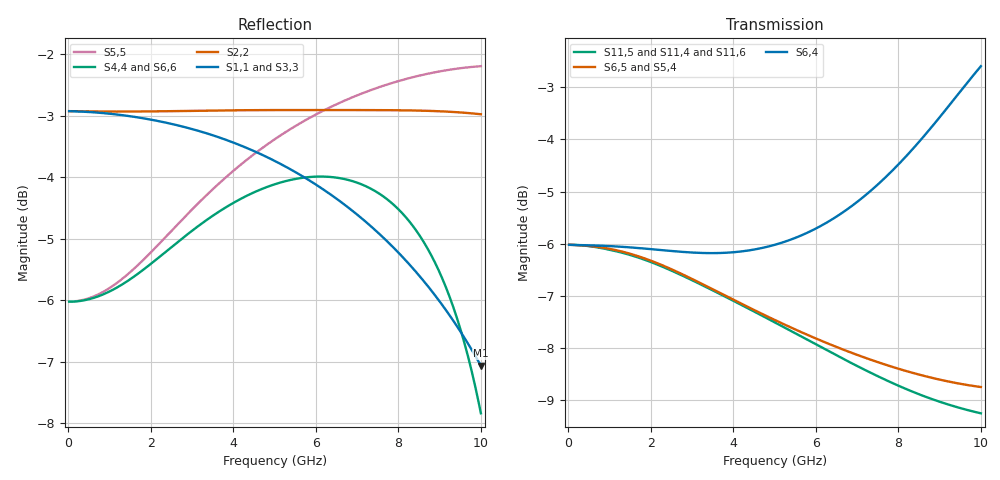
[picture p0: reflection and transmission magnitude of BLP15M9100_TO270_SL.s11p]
! Touchstone file from project BLP15M9100_TO270
! Exported from HFSS 2017.2.0
! Variables:
!  AirBox_H = 20mm
!  AirBox_L = 30mm
!  AirBox_W = 60mm
!  pcb_h = 502um
# GHZ S MA R 50.000000
! Terminal data exported
! Port[1] = P1_BWT4_13_Rect_T1
! Port[2] = P2_BWT10_13_Rect_T1
! Port[3] = P3_BWT6_13_Rect_T1
! Port[4] = P4_BWT1_Rect_T1
! Port[5] = P5_BWT11_Rect_T1
! Port[6] = P6_BWT7_Rect_T1
! Port[7] = P15_BWT14_Rect_T1
! Port[8] = P16_BWT14_Rect_T1
! Port[9] = P17_BWT14_Rect_T1
! Port[10] = Box3_T1
! Port[11] = Box2_T1
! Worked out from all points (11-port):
!   450 points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, 22.22 MHz to 10 GHz, reference per port
!   strongest paths, dB at 22.22 MHz, 2.511 GHz, 5.022 GHz, 7.511 GHz, 10 GHz:
!     S6,4: -6.0, -6.1, -6.0, -4.9, -2.6
!     S6,5: -6.0, -6.5, -7.5, -8.3, -8.8
!     S5,4: -6.0, -6.5, -7.5, -8.3, -8.7
!     S11,5: -6.0, -6.5, -7.5, -8.5, -9.3
!     S11,4: -6.0, -6.5, -7.5, -8.6, -9.3
!     S11,6: -6.0, -6.5, -7.6, -8.6, -9.4
!   lowest |S11| = -7.1 dB at 10 GHz (marker M1), VSWR 2.59
!   |S11| at or under -10 dB: nowhere
